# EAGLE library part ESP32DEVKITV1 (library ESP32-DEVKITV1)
https://github.com/shridattdudhat
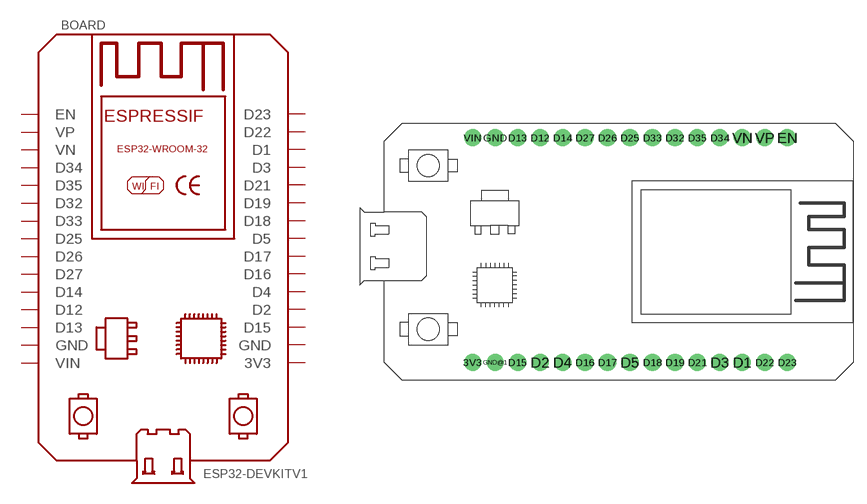
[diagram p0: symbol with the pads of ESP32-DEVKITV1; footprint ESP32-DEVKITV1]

Designator prefix BOARD

## ESP32DEVKITV1, ESP32DEVKITV1SHRIDATTDUDHAT  [ESP32-DEVKITV1]
3V3  3V3
D1  D1
D2  D2
D3  D3
D4  D4
D5  D5
D12  D12
D13  D13
D14  D14
D15  D15
D16  D16
D17  D17
D18  D18
D19  D19
D21  D21
D22  D22
D23  D23
D25  D25
D26  D26
D27  D27
D32  D32
D33  D33
D34  D34
D35  D35
EN  EN
GND  GND
GND@1  GND
VIN  VIN
VN  VN
VP  VP

## Footprint ESP32-DEVKITV1 (pad centres in mm)
drill 1 pad 1.93: 3V3 0,0; D1 30.48,0; D2 7.62,0; D3 27.94,0; D4 10.16,0; D5 17.78,0; D12 7.62,25.4; D13 5.08,25.4; D14 10.16,25.4; D15 5.08,0; D16 12.7,0; D17 15.24,0; D18 20.32,0; D19 22.86,0; D21 25.4,0; D22 33.02,0; D23 35.56,0; D25 17.78,25.4; D26 15.24,25.4; D27 12.7,25.4; D32 22.86,25.4; D33 20.32,25.4; D34 27.94,25.4; D35 25.4,25.4; EN 35.56,25.4; GND 2.54,25.4; GND@1 2.54,0; VIN 0,25.4; VN 30.48,25.4; VP 33.02,25.4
